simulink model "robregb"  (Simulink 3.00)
settings: Solver=ode5  StartTime=0.0  StopTime=15  FixedStep=10e-5  RelTol=1e-6  AbsTol=1e-6
libraries: simulink3 x5

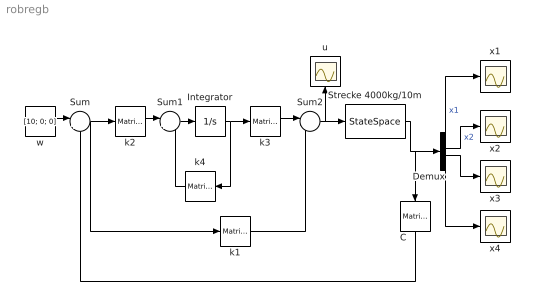
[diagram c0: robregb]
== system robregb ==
  C : simulink3/Math/Matrix Gain  Orientation=down  K=[1 0 0 0;0 1 0 0;0 0 1 0]
  Demux : Demux  Outputs=4
  Integrator : Integrator  ExternalReset=none  InitialConditionSource=internal  InitialCondition=0  LimitOutput=off  UpperSaturationLimit=inf  LowerSaturationLimit=-inf  ShowSaturationPort=off  ShowStatePort=off  AbsoluteTolerance=auto
  Strecke 4000kg/10m : StateSpace  A=[0 1 0 0;0 0 39.24 0;0 0 0 1;0 0 -4.905 0]  B=[0;0.001;0; -0.0001]  C=[1 0 0 0;0 1 0 0;0 0 1 0;0 0 0 1]  D=[0;0;0;0]  X0=[0;0;0;0]
  Sum : Sum  Inputs=|+-  SaturateOnIntegerOverflow=on
  Sum1 : Sum  Inputs=|+-  SaturateOnIntegerOverflow=on
  Sum2 : Sum  Inputs=|-+  SaturateOnIntegerOverflow=on
  k1 : simulink3/Math/Matrix Gain  K=[144.675 10294.8 -10032.5]
  k2 : simulink3/Math/Matrix Gain  K=[7.244 25.353 -306.174]
  k3 : simulink3/Math/Matrix Gain  K=-1000.68
  k4 : simulink3/Math/Matrix Gain  Orientation=left  K=0.625
  u : Scope
  w : Constant  Value=[10; 0; 0]
  x{1..4} (4 alike) : Scope
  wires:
  w/1 -> Sum/1
  k2/1 -> Sum1/1
  Sum1/1 -> Integrator/1
  k3/1 -> Sum2/1
  Sum2/1 -> Strecke 4000kg/10m/1, u/1
  Demux/3 -> x3/1
  Demux/4 -> x4/1
  Demux/1 -> x1/1  "x1"
  Demux/2 -> x2/1  "x2"
  Strecke 4000kg/10m/1 -> Demux/1, C/1
  C/1 -> Sum/2
  Sum/1 -> k2/1, k1/1
  k1/1 -> Sum2/2
  k4/1 -> Sum1/2
  Integrator/1 -> k3/1, k4/1
